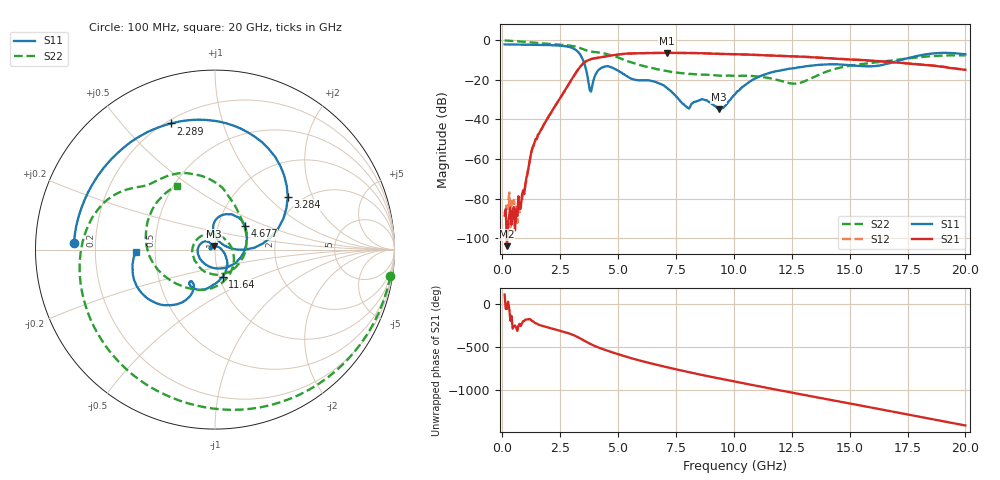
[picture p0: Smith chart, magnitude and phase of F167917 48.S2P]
!  2-Port S-parameters saved by WinCal
! VAR MeasName=S-Parameters (CALIBRATED_DATA) read from VNA (N5242A)
! VAR MeasDate=2016-11-22 9:02:11
! VAR NAME=F167917 48
! VAR FILENAME=F167917 48.S2P
! VAR DATE=2016-11-22 9:02:11
! VAR PHYS_PORTS=1,2
# Hz S DB R 50
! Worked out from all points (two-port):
!   401 points, 100 MHz to 20 GHz, reference 50 ohm
!   highest |S21| = -6.36 dB at 7.115 GHz (marker M1); lowest = -104.0 dB at 199.5 MHz (marker M2)
!   |S21| within 3 dB of the highest: 3.897 GHz to 14.46 GHz (10.56 GHz wide, 115 % of centre)
!   lowest |S11| = -34.8 dB at 9.354 GHz (marker M3), VSWR 1.04, Z = 49.5 + j1.73 ohm
!   |S11| at or under -10 dB: 3.486 GHz to 17.21 GHz (13.72 GHz wide, 133 % of centre)
!   |S22| runs from -21.9 to -0.1 dB; largest |S21 - S12| = 0.0061
!   S11 on the Smith chart (normalised r, x): 100 MHz: 0.12, +0.02; 2.289 GHz: 0.22, +0.69; 3.284 GHz: 1.70, +1.34; 4.677 GHz: 1.34, +0.37; 11.64 GHz: 1.04, -0.32; 20 GHz: 0.39, -0.01
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1e8  -2.09 177.3  -88.45 108.9  -87.37 -129.8  -0.10 -8.7
1.995e8  -2.10 174.7  -103.97 -57.6  -82.16 127.4  -0.16 -16.9
8.4625e8  -2.19 157.4  -78.37 132.5  -80.97 155.7  -0.68 -66.9
1.34375e9  -2.28 143.3  -53.32 156.1  -53.47 154.0  -1.22 -100.1
2.289e9  -2.56 109.3  -33.07 64.5  -33.04 64.3  -2.02 -152.6
3.284e9  -6.00 35.9  -14.63 -26.9  -14.64 -26.9  -3.60 155.0
3.43325e9  -8.64 18.3  -12.46 -48.8  -12.46 -48.7  -4.27 147.9
3.83125e9  -25.93 64.8  -9.54 -106.8  -9.52 -106.8  -5.71 135.7
4.1795e9  -14.78 84.0  -8.77 -146.9  -8.74 -147.0  -6.19 123.8
4.677e9  -13.52 38.2  -7.72 166.3  -7.72 166.2  -7.47 102.1
5.62225e9  -19.61 -88.3  -6.65 88.0  -6.62 87.9  -11.37 65.9
6.7665e9  -21.68 152.0  -6.39 9.5  -6.39 9.3  -14.82 14.9
7.11475e9  -24.09 133.8  -6.36 -12.6  -6.37 -12.6  -15.55 -7.4
7.9605e9  -33.61 148.1  -6.45 -63.4  -6.45 -63.5  -16.89 -68.0
9.3535e9  -34.82 106.0  -6.86 -142.0  -6.87 -142.1  -17.84 -139.0
1.005e10  -27.33 -9.7  -7.03 -179.4  -7.05 -179.2  -17.96 -160.7
1.1642e10  -16.13 -73.8  -7.71 97.8  -7.68 97.9  -19.35 135.8
1.338325e10  -12.75 -105.4  -8.58 8.9  -8.53 9.0  -18.98 -21.3
1.51245e10  -12.75 -128.0  -9.78 -77.7  -9.74 -77.9  -12.64 -106.0
1.67165e10  -11.62 -118.1  -10.90 -158.9  -10.88 -158.9  -10.35 -146.3
1.8408e10  -6.92 -140.0  -12.68 114.9  -12.51 114.2  -8.16 170.7
2e10  -7.10 -178.5  -14.92 33.7  -14.85 32.9  -7.67 120.7
